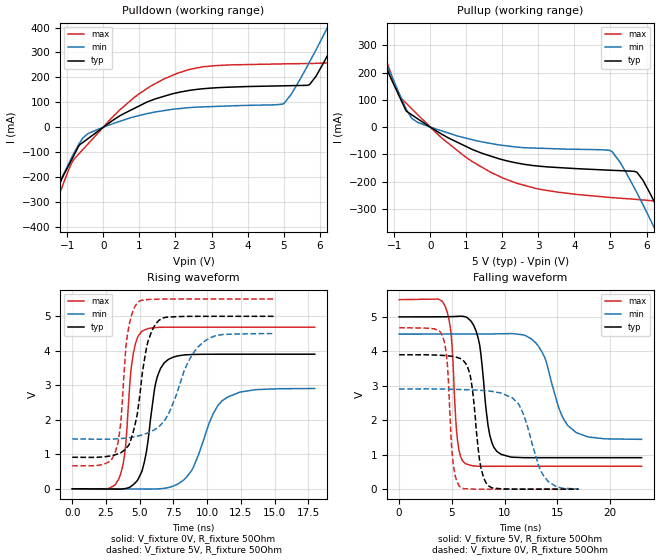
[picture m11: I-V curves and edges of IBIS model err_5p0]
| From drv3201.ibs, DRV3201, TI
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|   err_5p0 Model
[Model]   err_5p0
Model_type   Output
Polarity   Non-Inverting
Vmeas = 2.5
Vref = 0
Cref = 2pF
Rref = 300
|   typ   min   max
|   (nom PVT)   (fast PVT)   (slow PVT)
C_comp   4.123e-12   3.961e-12   4.552e-12
| Where nom  PVT is Nominal Process, 5V, 27C
|   Fast PVT is Strong Process,  5.5V, -40C
|   Slow PVT is Weak Process,   4.5V, 150C
[Voltage Range]   5   4.5   5.5
|Junction Temperature
[Temperature Range]   27   150   -40
[Pullup Reference]   5   4.5   5.5
[Pulldown Reference]   0   0   0
[Power Clamp Reference]   5   4.5   5.5
[GND Clamp Reference]   0   0   0
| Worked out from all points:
|   slope of the pulldown table from 0 to 0.75 V, typ, clamps not added: 11.1 ohm
|   slope of the pullup table from 0 to 0.75 V, typ, clamps not added: 13.6 ohm
|   falling waveform, V_fixture 5V, R_fixture 50Ohm: 20-80 % time 866ps typ, 1.87ns min, 550ps max; typ from 5 V to 0.914 V
|   rising waveform, V_fixture 0V, R_fixture 50Ohm: 20-80 % time 874ps typ, 1.74ns min, 601ps max; typ from 0 V to 3.9 V
|   rising waveform, V_fixture 5V, R_fixture 50Ohm: 20-80 % time 985ps typ, 1.94ns min, 618ps max; typ from 0.914 V to 5 V
|   falling waveform, V_fixture 0V, R_fixture 50Ohm: 20-80 % time 824ps typ, 1.8ns min, 528ps max; typ from 3.9 V to 0 V
[Pulldown]
|   Voltage   I(typ)   I(min)   I(max)
-5V       -1.564A    -1.414A    -1.724A
-2.844V   -801.8mA   -722.4mA   -898.6mA
-1.375V   -282.9mA   -267.1mA   -326.5mA
-841.5mV  -119.7mA   -110.7mA   -134mA
-427.5mV  -46.2mA    -26.11mA   -67.41mA
863.5mV   75.69mA    41.89mA    120.2mA
2.051V    138.4mA    73.7mA     216.3mA
5.013V    166mA      96.02mA    254.1mA
5.72V     170.9mA    262.1mA    255.3mA
6.303V    311.4mA    424.2mA    258.4mA
6.891V    480.3mA    590.7mA    403.2mA
10V       1.469A     1.521A     1.429A
[Pullup]
|   Voltage   I(typ)   I(min)   I(max)
-5V       1.553A     1.452A     1.681A
-2.795V   773.3mA    730mA      842.4mA
-1.375V   273.1mA    276.8mA    302.4mA
-907.5mV  126.7mA    137.1mA    130.7mA
-513mV    45.04mA    32.06mA    67.37mA
968mV     -69.24mA   -39.56mA   -108.5mA
2.376V    -130.8mA   -72.78mA   -204.6mA
5.04V     -158.2mA   -89.55mA   -258.2mA
5.735V    -165.5mA   -241.2mA   -264.8mA
6.303V    -297.3mA   -392.6mA   -271.6mA
6.835V    -448.1mA   -537.1mA   -399.7mA
10V       -1.469A    -1.482A    -1.471A
[Ramp]
R_load = 50
|   typ   min   max
dV/dt_r   2.34058/8.70464e-10   1.74417/1.72866e-09   2.81133/5.94833e-10
dV/dt_f   2.45167/8.57523e-10   1.83305/1.85677e-09   2.90159/5.40044e-10
[Falling Waveform]
V_fixture = 5V
V_fixture_min = 4.5V
V_fixture_max = 5.5V
R_fixture = 50Ohm
|   Time   V(typ)   V(min)   V(max)
0s        5V         4.5V       5.5V
4.392ns   5.004V     4.501V     5.29V
4.94ns    5.008V     4.501V     4.454V
5.528ns   5.015V     4.501V     1.425V
6.308ns   5V         4.501V     735mV
7.486ns   4.386V     4.502V     665mV
9.252ns   1.097V     4.507V     663.3mV
13.23ns   913.4mV    4.138V     664mV
16.78ns   913.9mV    1.642V     664mV
22.98ns   913.9mV    1.445V     664mV
[Rising Waveform]
V_fixture = 0V
V_fixture_min = 0V
V_fixture_max = 0V
R_fixture = 50Ohm
|   Time   V(typ)   V(min)   V(max)
0s        587.9pV    150nV      435.5pV
3.44ns    -10.87mV   -2.196mV   277.4mV
3.954ns   9.409mV    -3.515mV   1.238V
4.528ns   120.6mV    -5.271mV   3.928V
5.178ns   521.3mV    -7.662mV   4.566V
6.194ns   3.079V     -5.703mV   4.675V
7.096ns   3.742V     31.98mV    4.685V
8.844ns   3.892V     524.2mV    4.686V
11.09ns   3.901V     2.546V     4.686V
17.98ns   3.901V     2.907V     4.686V
[Rising Waveform]
V_fixture = 5V
V_fixture_min = 4.5V
V_fixture_max = 5.5V
R_fixture = 50Ohm
|   Time   V(typ)   V(min)   V(max)
0s        913.9mV    1.445V     664mV
3.17ns    983.8mV    1.444V     1.029V
3.578ns   1.039V     1.454V     1.868V
4.084ns   1.214V     1.474V     4.45V
4.982ns   2.626V     1.54V      5.441V
5.614ns   4.273V     1.62V      5.487V
6.454ns   4.891V     1.809V     5.499V
8.586ns   4.998V     3.673V     5.5V
9.728ns   5V         4.257V     5.5V
14.98ns   5V         4.5V       5.5V
[Falling Waveform]
V_fixture = 0V
V_fixture_min = 0V
V_fixture_max = 0V
R_fixture = 50Ohm
|   Time   V(typ)   V(min)   V(max)
0s        3.901V     2.907V     4.686V
4.122ns   3.882V     2.906V     4.433V
4.598ns   3.871V     2.902V     3.52V
5.144ns   3.849V     2.898V     684.3mV
5.794ns   3.789V     2.892V     62.78mV
6.714ns   3.334V     2.882V     6.204mV
7.6ns     888.4mV    2.87V      -315.2uV
8.498ns   91.87mV    2.849V     -296.3uV
14.16ns   -12.73uV   214.5mV    3.621nV
17ns      357.2nV    7.375mV    57.12nV
